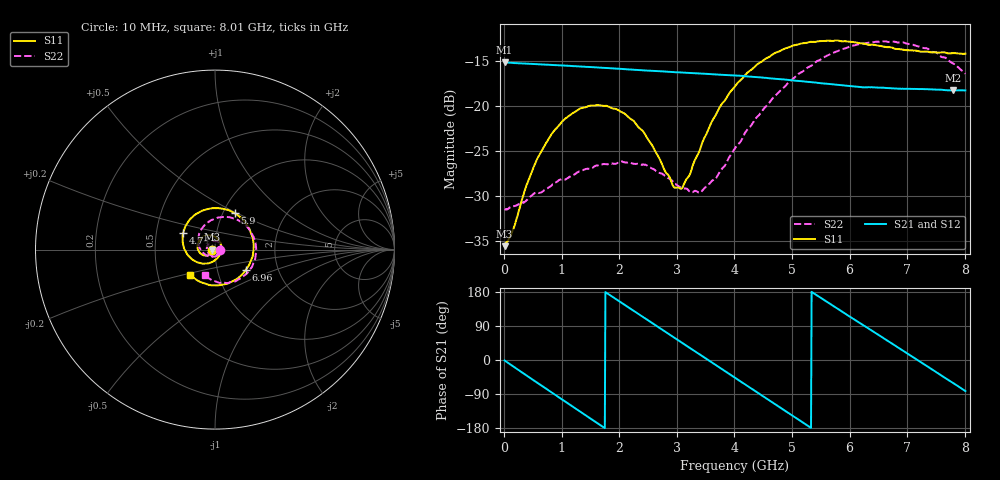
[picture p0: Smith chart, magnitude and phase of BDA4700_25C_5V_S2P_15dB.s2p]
!Agilent Technologies,E5071B,MY42404982,A.09.10
!Date: Mon Oct 20 13:33:43 2025
!Data & Calibration Information:
!Freq	S11:SOLT2(ON)	S21:SOLT2(ON)	S12:SOLT2(ON)	S22:SOLT2(ON)
# Hz S RI R 50
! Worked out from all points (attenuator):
!   801 points, 10 MHz to 8.01 GHz, reference 50 ohm
!   highest |S21| = -15.10 dB at 10 MHz (marker M1); lowest = -18.2 dB at 7.8 GHz (marker M2)
!   lowest |S11| = -35.6 dB at 10 MHz (marker M3), VSWR 1.03, Z = 48.4 - j0.112 ohm
!   |S11| at or under -10 dB: start of sweep to end of sweep
!   |S22| runs from -31.5 to -12.8 dB; largest |S21 - S12| = 0.0013
!   S11 on the Smith chart (normalised r, x): 10 MHz: 0.97, -0.00; 4.74 GHz: 0.69, +0.13; 5.9 GHz: 1.14, +0.49; 6.96 GHz: 1.38, -0.32; 8.01 GHz: 0.73, -0.21
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1e7  -0.0165 -0.00116  0.1758 -0.00382  0.1757 -0.00405  0.0266 -0.00102
1.5e8  -0.0177 -0.00966  0.1676 -0.0478  0.1676 -0.0479  0.0265 -0.0077
3.9e8  -0.0265 -0.0246  0.1309 -0.1129  0.1307 -0.1131  0.0205 -0.0217
6.3e8  -0.0434 -0.0332  0.0711 -0.1559  0.0709 -0.1559  0.00904 -0.0317
1.01e9  -0.0788 -0.0234  -0.0422 -0.1634  -0.0422 -0.1634  -0.0199 -0.0336
1.35e9  -0.0974 0.0087  -0.1259 -0.1088  -0.126 -0.1089  -0.0415 -0.0135
1.72e9  -0.0857 0.0525  -0.1635 -0.00903  -0.1636 -0.00905  -0.0437 0.0185
2.09e9  -0.046 0.0785  -0.1331 0.0907  -0.1332 0.0908  -0.0222 0.0433
2.68e9  0.0252 0.0457  0.00978 0.1566  0.00972 0.1565  0.0265 0.0333
2.95e9  0.0347 0.00627  0.079 0.1333  0.0789 0.1332  0.0353 0.0121
3.09e9  0.0313 -0.0153  0.1085 0.1096  0.108 0.1098  0.0349 -0.00142
3.43e9  -0.00274 -0.0609  0.1492 0.03  0.1493 0.0299  0.0164 -0.0292
4.01e9  -0.1122 -0.0636  0.1017 -0.1082  0.1017 -0.108  -0.0484 -0.0321
4.74e9  -0.1772 0.0929  -0.0714 -0.1228  -0.0712 -0.1231  -0.0916 0.0728
5.35e9  -0.0615 0.2201  -0.136 0.00259  -0.136 0.00225  -0.00581 0.1693
5.9e9  0.1111 0.2019  -0.0741 0.1077  -0.0743 0.1074  0.1338 0.161
6.26e9  0.1907 0.1155  0.000161 0.1274  0.00127 0.1273  0.2055 0.0884
6.68e9  0.2119 -0.0252  0.0833 0.0947  0.0835 0.0948  0.2267 -0.0292
6.96e9  0.173 -0.1114  0.1163 0.0461  0.1165 0.0456  0.1994 -0.1055
7.37e9  0.0604 -0.1919  0.1176 -0.04  0.1176 -0.0401  0.1083 -0.1778
7.8e9  -0.0822 -0.1802  0.0592 -0.1071  0.059 -0.1075  -0.0123 -0.1724
8.01e9  -0.1372 -0.1407  0.0169 -0.1213  0.0171 -0.1215  -0.0576 -0.1406
